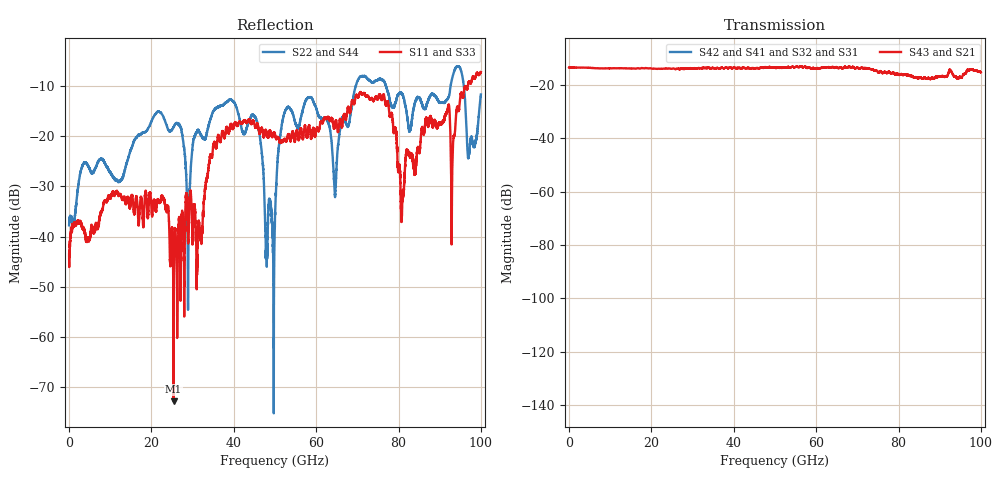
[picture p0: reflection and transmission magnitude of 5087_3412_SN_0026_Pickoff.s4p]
! Created Mon Apr 13 10:49:21 2009
# Hz S  RI  R 50
! 4 Port Network Data from SP1.SP block
! freq  magS11  angS11  magS12  angS12  magS13  angS13  magS14  angS14
!  magS21  angS21  magS22  angS22  magS23  angS23  magS24  angS24
!  magS31  angS31  magS32  angS32  magS33  angS33  magS34  angS34
!  magS41  angS41  magS42  angS42  magS43  angS43  magS44  angS44
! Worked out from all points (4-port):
!   10000 points, 10 MHz to 100 GHz, reference 50 ohm
!   strongest paths, dB at 10 MHz, 25.01 GHz, 50.01 GHz, 75.01 GHz, 100 GHz:
!     S43: -13.5, -14.0, -13.6, -15.3, -15.3
!     S21: -13.5, -14.0, -13.6, -15.3, -15.3
!     S42: -, -, -, -, -
!     S41: -, -, -, -, -
!     S32: -, -, -, -, -
!     S31: -, -, -, -, -
!   lowest |S11| = -72.8 dB at 25.37 GHz (marker M1), VSWR 1.00, Z = 50 + j0.0131 ohm
!   |S11| at or under -10 dB: start of sweep to 96.18 GHz; 96.19 GHz to 96.83 GHz (640.1 MHz wide, 0.663 % of centre)
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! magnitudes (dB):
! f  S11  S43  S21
! 10 MHz  -43.6  -13.5  -13.5
! 25.37 GHz  -72.8  -13.9  -13.9
! 44.98 GHz  -17.5  -13.9  -13.9
! 49.57 GHz  -19.6  -13.5  -13.5
! 53 GHz  -20.3  -13.4  -13.4
! 80.94 GHz  -32.8  -16.2  -16.2
! 100 GHz  -7.2  -15.3  -15.3
